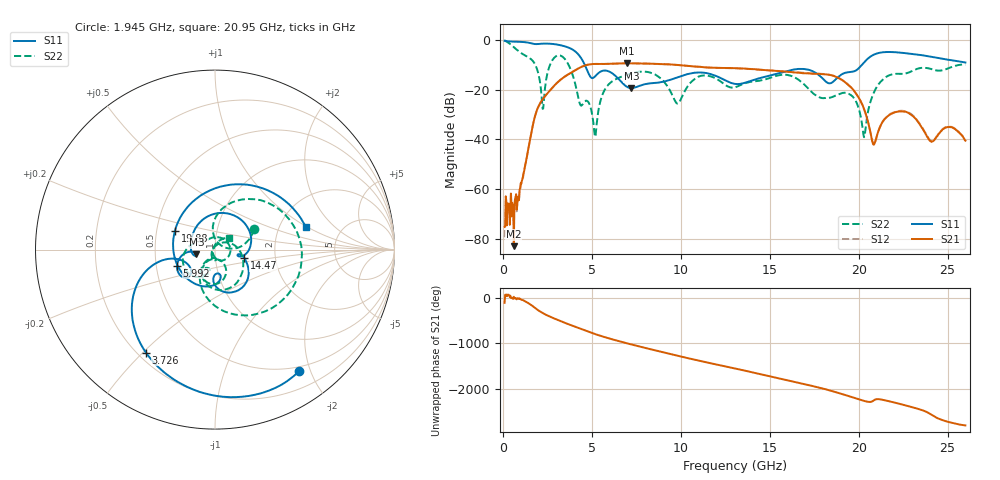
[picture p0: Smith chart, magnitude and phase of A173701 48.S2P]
!  2-Port S-parameters saved by WinCal
! VAR MeasName=S-Parameters (CALIBRATED_DATA) read from VNA (N5245A)
! VAR MeasDate=2017-6-7 10:31:36
! VAR NAME=A173701 48
! VAR FILENAME=A173701 48.S2P
! VAR DATE=2017-6-7 10:31:36
! VAR PHYS_PORTS=1,2
# Hz S DB R 50
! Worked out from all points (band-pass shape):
!   801 points, 100 MHz to 26 GHz, reference 50 ohm
!   highest |S21| = -9.43 dB at 6.996 GHz (marker M1); lowest = -83.0 dB at 618 MHz (marker M2)
!   |S21| within 3 dB of the highest: 4.023 GHz to 15.3 GHz (11.27 GHz wide, 117 % of centre)
!   lowest |S11| = -19.4 dB at 7.223 GHz (marker M3), VSWR 1.24, Z = 40.6 - j2.22 ohm
!   |S11| at or under -10 dB: 4.603 GHz to 20.19 GHz (15.59 GHz wide, 126 % of centre)
!   |S22| runs from -39.1 to -0.2 dB; largest |S21 - S12| = 0.0054
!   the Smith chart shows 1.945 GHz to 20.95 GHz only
!   S11 on the Smith chart (normalised r, x): 1.945 GHz: 0.44, -1.83; 3.726 GHz: 0.23, -0.51; 5.992 GHz: 0.64, -0.12; 14.47 GHz: 1.38, -0.14; 19.88 GHz: 0.62, +0.14; 20.95 GHz: 2.79, +0.98
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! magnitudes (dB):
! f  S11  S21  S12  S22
! 100 MHz  -0.3  -75.2  -79.4  -0.2
! 618 MHz  -0.7  -83.0  -73.9  -2.9
! 1.945 GHz  -1.7  -27.7  -27.7  -12.3
! 2.269 GHz  -1.5  -23.6  -23.6  -27.6
! 2.884 GHz  -1.7  -18.5  -18.5  -7.2
! 3.726 GHz  -3.2  -13.7  -13.6  -10.5
! 4.438 GHz  -7.8  -10.8  -10.8  -26.3
! 5.183 GHz  -14.7  -9.7  -9.7  -39.0
! 5.992 GHz  -12.8  -9.6  -9.6  -17.6
! 6.996 GHz  -19.0  -9.4  -9.4  -14.0
! 7.223 GHz  -19.4  -9.4  -9.4  -13.5
! 8.744 GHz  -17.2  -9.7  -9.7  -14.8
! 9.812 GHz  -15.1  -10.1  -10.1  -25.6
! 11.11 GHz  -13.1  -10.8  -10.9  -14.5
! 13.05 GHz  -17.7  -11.4  -11.4  -19.1
! 14.47 GHz  -15.3  -12.0  -12.0  -16.4
! 17.39 GHz  -12.5  -13.6  -13.5  -21.1
! 19.88 GHz  -12.1  -21.9  -21.9  -25.2
! 20.33 GHz  -8.8  -28.4  -28.5  -38.8
! 20.95 GHz  -5.7  -40.5  -40.7  -19.8
! 21.69 GHz  -4.9  -30.3  -30.2  -14.3
! 26 GHz  -9.1  -40.5  -40.6  -10.0
